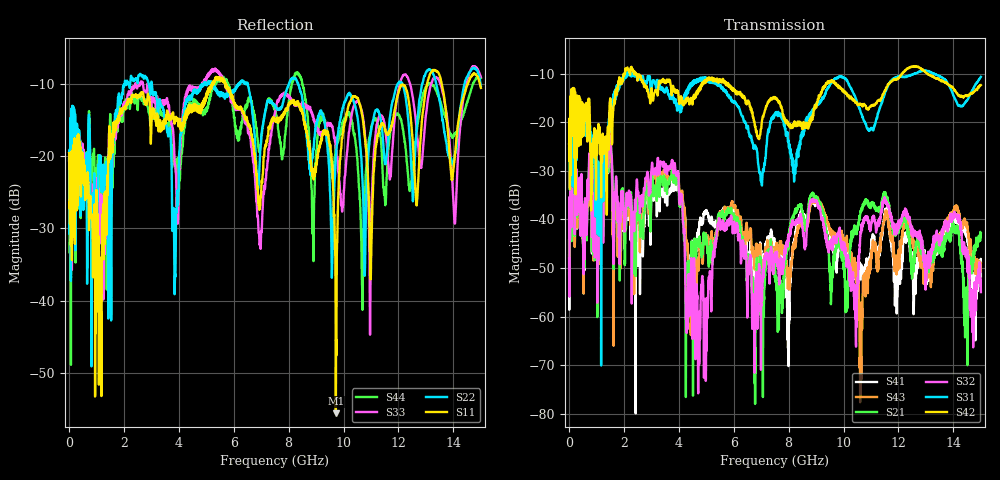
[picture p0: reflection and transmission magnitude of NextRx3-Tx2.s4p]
! FILE: N:\QM 2007\Prüfprotokolle\Highspeed\Konfektionierte Ltg\L45593-D106\D30\8216\0002\Next  Platine 2\NextRx3-Tx2.s4p
# MHz S DB R 50.00
! FREQ  S11  S12  S13  S14
!  S21  S22  S23  S24
!  S31  S32  S33  S34
!  S41  S42  S43  S44
!  DB  ANG  DB  ANG  DB  ANG  DB  ANG
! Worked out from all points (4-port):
!   2999 points, 10 MHz to 15 GHz, reference 50 ohm
!   strongest paths, dB at 10 MHz, 3.755 GHz, 7.505 GHz, 11.26 GHz, 15 GHz:
!     S42: -24.6, -13.5, -14.9, -15.6, -12.3
!     S31: -25.4, -15.2, -18.4, -18.1, -10.6
!     S32: -48.0, -27.8, -46.8, -40.9, -55.0
!     S21: -51.1, -30.1, -49.6, -38.2, -42.8
!     S43: -47.3, -29.8, -46.3, -48.3, -48.9
!     S41: -44.3, -32.3, -45.7, -45.6, -51.7
!   lowest |S11| = -55.6 dB at 9.72 GHz (marker M1), VSWR 1.00, Z = 49.8 - j0.0358 ohm
!   |S11| at or under -10 dB: start of sweep to 5.212 GHz; 5.698 GHz to 13.04 GHz (7.343 GHz wide, 78.4 % of centre); 13.58 GHz to 14.52 GHz (948.1 MHz wide, 6.75 % of centre)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
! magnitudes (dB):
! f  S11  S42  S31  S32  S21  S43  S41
! 10 MHz  -19.6  -24.6  -25.4  -48.0  -51.1  -47.3  -44.3
! 1.5 GHz  -20.4  -15.4  -20.1  -21.8  -21.6  -22.4  -22.2
! 2.37 GHz  -11.7  -10.0  -10.2  -40.2  -40.5  -54.3  -44.3
! 3.915 GHz  -14.9  -13.9  -16.3  -31.0  -32.4  -31.8  -34.0
! 4.675 GHz  -13.5  -14.1  -11.5  -55.7  -45.1  -48.2  -42.7
! 9.72 GHz  -55.6  -12.0  -11.0  -44.6  -46.6  -44.2  -49.5
! 15 GHz  -10.6  -12.3  -10.6  -55.0  -42.8  -48.9  -51.7
